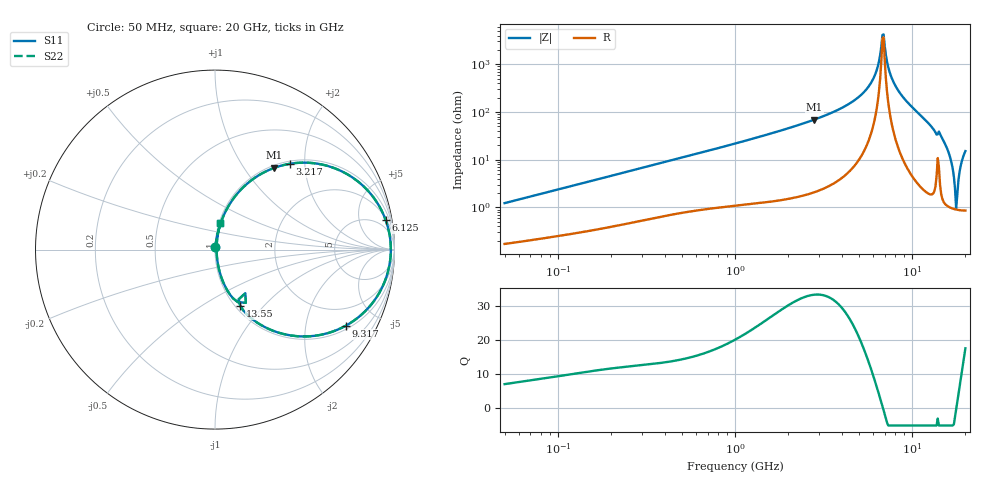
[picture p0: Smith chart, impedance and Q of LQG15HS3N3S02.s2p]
!Murata Part Number: LQG15HS3N3S02
!These Parameters are Measured in Series Mode Connection
!  o--[Z]--o
!Port1  Port2
!  o-------o
!Freq. Start=50[MHz] Stop=20[GHz], 401[Steps]
# Hz S RI R 50
!Freq.(Hz) S11(Real) S11(Imag) S21(Real) S21(Imag) S12(Real) S12(Imag) S22(Real) S22(Imag)
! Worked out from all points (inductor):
!   401 points, 50 MHz to 20 GHz, reference 50 ohm
!   read as one part in series: L = 3.84 nH near 51.52 MHz
!   highest Q = 33.2 at 2.811 GHz (marker M1), where L = 3.93 nH
!   self-resonance near 6.802 GHz
!   S11 on the Smith chart (normalised r, x): 50 MHz: 1.00, +0.02; 3.217 GHz: 1.05, +1.68; 6.125 GHz: 2, +11; 9.317 GHz: 1.14, -3.34; 13.55 GHz: 1.05, -0.75; 20 GHz: 1.02, +0.30
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5e7  0.00187 0.0122  0.9981 -0.0122  0.9981 -0.0122  0.00187 0.0122
1.364002e8  0.00403 0.0316  0.996 -0.0316  0.996 -0.0316  0.00403 0.0316
3.721004e8  0.013 0.0815  0.987 -0.0815  0.987 -0.0815  0.013 0.0815
1e9  0.0546 0.2037  0.9454 -0.2037  0.9454 -0.2037  0.0546 0.2037
2.728004e9  0.3136 0.4491  0.6864 -0.4491  0.6864 -0.4491  0.3136 0.4491
2.810964e9  0.3305 0.4556  0.6695 -0.4556  0.6695 -0.4556  0.3305 0.4556
3.216634e9  0.4168 0.4781  0.5832 -0.4781  0.5832 -0.4781  0.4168 0.4781
4.89267e9  0.7794 0.3925  0.2206 -0.3925  0.2206 -0.3925  0.7794 0.3925
6.125241e9  0.9507 0.1655  0.0493 -0.1655  0.0493 -0.1655  0.9507 0.1655
6.802353e9  0.9796 0.0122  0.0204 -0.0122  0.0204 -0.0122  0.9796 0.0122
7.009217e9  0.9785 -0.0349  0.0215 0.0349  0.0215 0.0349  0.9785 -0.0349
7.442007e9  0.9618 -0.1303  0.0382 0.1303  0.0382 0.1303  0.9618 -0.1303
8.141811e9  0.8991 -0.2673  0.1009 0.2673  0.1009 0.2673  0.8991 -0.2673
9.316812e9  0.7278 -0.4246  0.2722 0.4246  0.2722 0.4246  0.7278 -0.4246
1.131968e10  0.3995 -0.4743  0.6005 0.4743  0.6005 0.4743  0.3995 -0.4743
1.354865e10  0.1406 -0.313  0.8594 0.313  0.8594 0.313  0.1406 -0.313
1.460232e10  0.1007 -0.2716  0.8993 0.2716  0.8993 0.2716  0.1007 -0.2716
1.597544e10  0.032 -0.1448  0.968 0.1448  0.968 0.1448  0.032 -0.1448
1.774144e10  0.00897 -0.00278  0.991 0.00278  0.991 0.00278  0.00897 -0.00278
1.828096e10  0.0101 0.0361  0.9899 -0.0361  0.9899 -0.0361  0.0101 0.0361
1.912117e10  0.0173 0.0923  0.9827 -0.0923  0.9827 -0.0923  0.0173 0.0923
2e10  0.0304 0.1455  0.9696 -0.1455  0.9696 -0.1455  0.0304 0.1455
